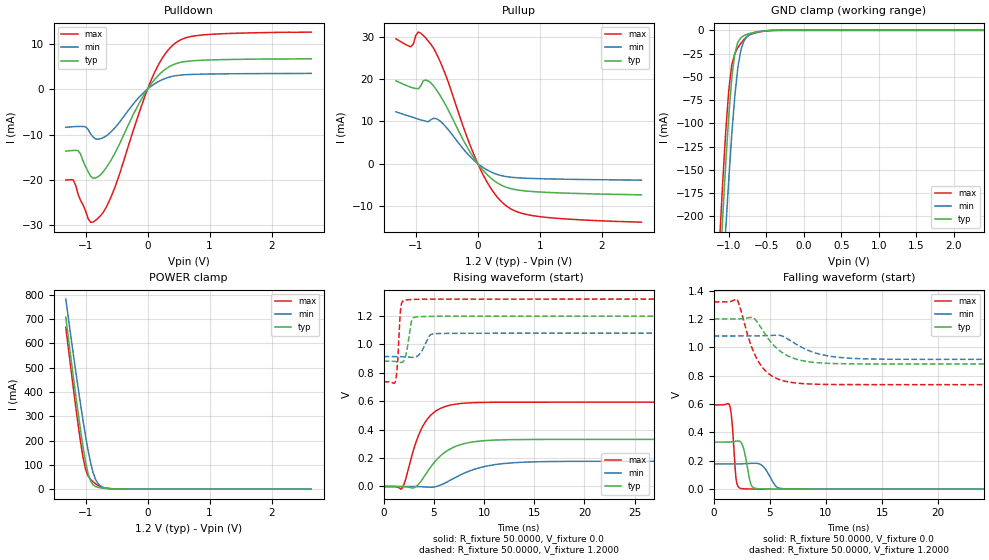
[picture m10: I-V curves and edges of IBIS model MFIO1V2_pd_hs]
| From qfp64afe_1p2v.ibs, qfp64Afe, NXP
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[Model] MFIO1V2_pd_hs
|   Model MFIO1V2_pd_hs
| This model was characterised for following simulation conditions:
| External (pad) voltage:
|   - Typ: 1.2V,   - Min: 1.08V,   - Max: 1.32V
| Library cells for typ/min/max conditions are connected as defined below:
|  IO - External Pad
|  A - Core Input
|  EN - Output Buffer Enable
|  BOOST - vdde
|  EHS - vdd
|  ENZI - vdd
|  EPD - vdd
|  EPUN - vdd
|  ZI - NC
|  ZIF - NC
|  gnd - gnd
|  gnde - gnde
|  vdd - vdd
|  vdde - vdde
| All other pins connected to ground
Model_type I/O
Polarity   Non-Inverting
Enable   Active-Low
Vinl =   0.3600V
Vinh =   0.8400V
Vmeas =  0.6000V
Cref =   20.0000F
Rref =   1.0000M
Vref =   0.0V
C_comp   1.6368pF   1.5495pF   1.7159pF
|C_comp_pullup   0.8309pF   0.8676pF   0.7830pF
|C_comp_pulldown   0.5929pF   0.6311pF   0.5574pF
[Model Spec]
| variable   typ   min   max
Vinh   0.3600V   0.3240V   0.3960V
Vinl   0.8400V   0.7560V   0.9240V
Vmeas   0.6000V   0.5400V   0.6600V
[Temperature Range]   25.0000   0.1250k   -40.0000
[Voltage Range]   1.2000V   1.0800V   1.3200V
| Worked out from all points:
|   slope of the pulldown table from 0 to 0.18 V, typ, clamps not added: 58.2 ohm
|   slope of the pullup table from 0 to 0.18 V, typ, clamps not added: 59.4 ohm
|   GND clamp passes 1 mA (typ) near -0.56 V on its own axis
|   POWER clamp passes 1 mA (typ) near -0.54 V on its own axis
|   rising waveform, R_fixture 50.0000, V_fixture 0.0: 20-80 % time 2.65ns typ, 3.73ns min, 1.92ns max; typ from 0 V to 0.331 V
|   rising waveform, R_fixture 50.0000, V_fixture 1.2000: 20-80 % time 420ps typ, 689ps min, 271ps max; typ from 0.882 V to 1.2 V
|   falling waveform, R_fixture 50.0000, V_fixture 0.0: 20-80 % time 470ps typ, 797ps min, 303ps max; typ from 0.331 V to 0 V
|   falling waveform, R_fixture 50.0000, V_fixture 1.2000: 20-80 % time 2.23ns typ, 2.81ns min, 1.78ns max; typ from 1.2 V to 0.882 V
[Pulldown]
|Voltage   I(typ)   I(min)   I(max)
-1.32V    -13.65mA   -8.413mA   -20.02mA
-1.2V     -13.51mA   -8.286mA   -20.01mA
-1.12V    -13.55mA   -8.228mA   -23.23mA
-920mV    -19.16mA   -9.85mA    -29.29mA
-720mV    -18.27mA   -10.7mA    -27.21mA
-520mV    -13.92mA   -8.406mA   -21.33mA
-160mV    -3.727mA   -2.148mA   -6.154mA
80mV      1.535mA    840.4uA    2.681mA
280mV     4.299mA    2.312mA    7.674mA
480mV     5.684mA    2.989mA    10.42mA
960mV     6.383mA    3.3mA      11.99mA
2.64V     6.67mA     3.446mA    12.53mA
[Pullup]
|Voltage   I(typ)   I(min)   I(max)
-1.32V    19.64mA    12.26mA    29.6mA
-1.08V    18.12mA    11.13mA    27.73mA
-960mV    17.74mA    10.54mA    31.21mA
-840mV    19.83mA    10.07mA    29.84mA
-720mV    18.57mA    10.71mA    27.56mA
-520mV    13.94mA    8.794mA    21.09mA
-200mV    4.663mA    2.883mA    7.362mA
40mV      -771.3uA   -452.7uA   -1.28mA
240mV     -3.804mA   -2.171mA   -6.507mA
480mV     -5.732mA   -3.143mA   -10.26mA
1.04V     -6.794mA   -3.614mA   -12.68mA
2.64V     -7.439mA   -3.951mA   -13.93mA
[GND_clamp]
|Voltage   I(typ)   I(min)   I(max)
-1.32V    -596.2mA   -647.7mA   -564.2mA
-1.12V    -261.7mA   -329.6mA   -222.8mA
-1.08V    -200.1mA   -270.2mA   -162.2mA
-1.04V    -142.4mA   -213.4mA   -108mA
-1V       -91.66mA   -160.1mA   -64.4mA
-960mV    -51.26mA   -111.8mA   -37.36mA
-920mV    -25.17mA   -71.04mA   -25.19mA
-880mV    -12.89mA   -40.68mA   -18.85mA
-800mV    -5.7mA     -11.79mA   -10.05mA
-680mV    -2.586mA   -2.926mA   -3.538mA
-440mV    -160.8uA   -186.1uA   -197.3uA
2.64V     0A         0A         0A
[POWER_clamp]
|Voltage   I(typ)   I(min)   I(max)
-1.32V    708.1mA    782.2mA    666.5mA
-1.2V     465.5mA    558mA      418.6mA
-1.12V    311.6mA    414.8mA    262.8mA
-1.04V    171.5mA    279.6mA    128.1mA
-1V       111.7mA    217mA      80.3mA
-960mV    64.07mA    159.3mA    53.87mA
-920mV    33.02mA    108.9mA    40.24mA
-880mV    17.44mA    68.44mA    30.42mA
-840mV    10.78mA    40.19mA    22.06mA
-760mV    5.295mA    13.21mA    9.362mA
-440mV    235.7uA    303.1uA    277.6uA
2.64V     0A         0A         0A
[Ramp]
| variable   typ   min   max
dV/dt_r  0.1989/2.6507n   0.1066/3.7290n   0.3561/1.9152n
dV/dt_f  0.1904/2.2327n   98.8032m/2.8148n   0.3496/1.7783n
R_load = 50.0000
[Rising Waveform]
R_fixture= 50.0000
V_fixture= 0.0
V_fixture_min= 0.0
V_fixture_max= 0.0
|time   V(typ)   V(min)   V(max)
0s        1.234nV    117.7nV    49.88pV
1.833ns   -130.6uV   80.57uV    -11.44mV
2.128ns   -1.644mV   80.34uV    36.36mV
3.412ns   11.58mV    -798.5uV   349.7mV
4.674ns   136.5mV    -5.414mV   500.9mV
6.05ns    238.5mV    22.16mV    561.2mV
7.96ns    300.6mV    92.12mV    586.1mV
11.31ns   327.4mV    156.2mV    593mV
16.57ns   331.4mV    175.7mV    593.6mV
100ns     331.4mV    177.7mV    593.5mV
[Rising Waveform]
R_fixture= 50.0000
V_fixture= 1.2000
V_fixture_min= 1.0800
V_fixture_max= 1.3200
|time   V(typ)   V(min)   V(max)
0s        882mV      914.8mV    736.7mV
1.165ns   880.1mV    915mV      739mV
1.36ns    877.5mV    915.2mV    846.4mV
1.737ns   872.7mV    913.9mV    1.273V
2.138ns   907.2mV    912mV      1.312V
2.496ns   1.041V     910.2mV    1.315V
2.963ns   1.188V     909mV      1.317V
4.598ns   1.198V     1.064V     1.319V
5.458ns   1.198V     1.077V     1.319V
100ns     1.199V     1.079V     1.319V
[Falling Waveform]
R_fixture= 50.0000
V_fixture= 0.0
V_fixture_min= 0.0
V_fixture_max= 0.0
|time   V(typ)   V(min)   V(max)
0s        331.4mV    177.7mV    593.5mV
1.419ns   331.8mV    177.7mV    588.1mV
1.619ns   333.7mV    177.6mV    483mV
2.015ns   338.8mV    177.5mV    57.64mV
2.605ns   300.6mV    178.8mV    2.748mV
3.317ns   32.38mV    182mV      1.003mV
4.194ns   1.977mV    172.8mV    421.3uV
5.596ns   579.7uV    16.49mV    123.7uV
6.706ns   264.8uV    1.638mV    49.86uV
100ns     2.827nV    122.2nV    7.767nV
[Falling Waveform]
R_fixture= 50.0000
V_fixture= 1.2000
V_fixture_min= 1.0800
V_fixture_max= 1.3200
|time   V(typ)   V(min)   V(max)
0s        1.199V     1.079V     1.319V
2.06ns    1.199V     1.079V     1.338V
3.45ns    1.211V     1.079V     986.9mV
4.249ns   1.132V     1.08V      866.7mV
4.96ns    1.05V      1.083V     809.1mV
5.932ns   971.6mV    1.083V     769.9mV
7.718ns   908.4mV    1.004V     745mV
10.46ns   885.9mV    935.5mV    737.6mV
15.36ns   882.2mV    915.8mV    736.6mV
100ns     882mV      914.8mV    736.7mV
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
